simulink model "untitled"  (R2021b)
settings: Solver=FixedStepDiscrete  StartTime=0.0  StopTime=inf  FixedStep=0.01  RelTol=1e-3
libraries: sculib x1, RS485_1_TxBytes_lib x1, RS485_2_TxBytes_lib x1

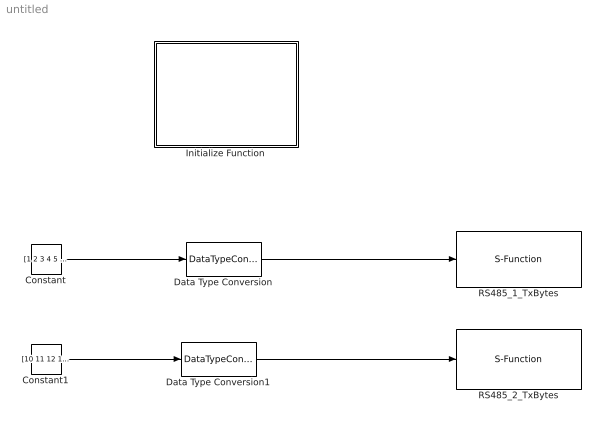
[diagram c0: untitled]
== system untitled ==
  Constant : Constant  Value=[1 2 3 4 5 6 7 8]
  Constant1 : Constant  Value=[10 11 12 13 14 15 16 17]
  Data Type Conversion : DataTypeConversion
  Data Type Conversion1 : DataTypeConversion
  Initialize Function : Subsystem  TreatAsAtomicUnit=on
  RS485_1_TxBytes : RS485_1_TxBytes_lib/S-Function  vu8=0
  RS485_2_TxBytes : RS485_2_TxBytes_lib/S-Function  vu8=0
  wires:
  Constant1/1 -> Data Type Conversion1/1
  Constant/1 -> Data Type Conversion/1
  Data Type Conversion/1 -> RS485_1_TxBytes/1
  Data Type Conversion1/1 -> RS485_2_TxBytes/1

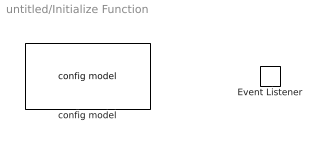
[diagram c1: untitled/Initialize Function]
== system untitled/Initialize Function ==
  Event Listener : EventListener  DisableCoverage=on  EventName=reset
  config model : sculib/SCU001/config model  Priority=0  iap=Uart2  uart1_baudrate=9600  uart2_baudrate=115200  rs485_1_baudrate=9600  rs485_2_baudrate=9600  rs485_1_read_interval=10  rs485_2_read_interval=10
